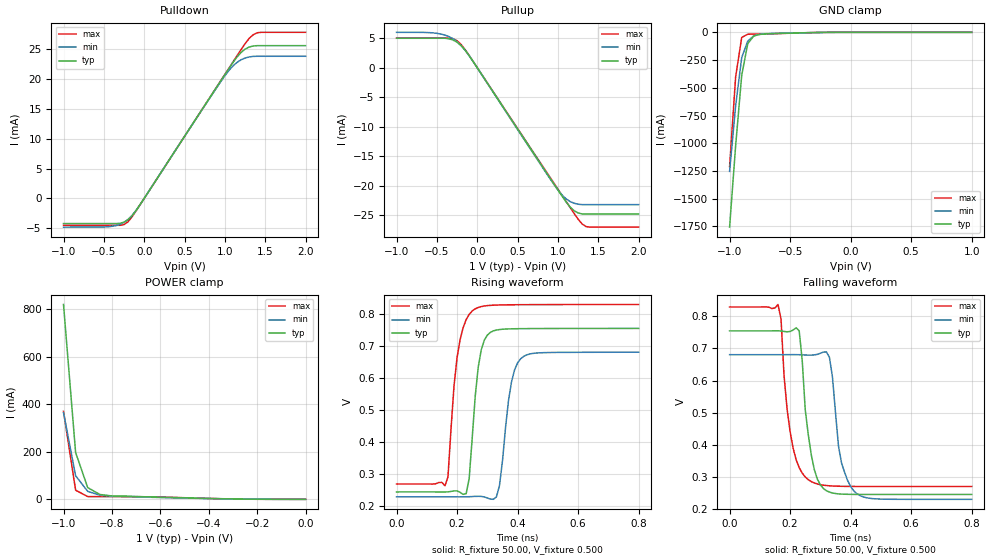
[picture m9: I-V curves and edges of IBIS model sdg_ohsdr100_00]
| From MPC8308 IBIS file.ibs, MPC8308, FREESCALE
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|Main and Boost models for Amp0: PCIx and SGMII protocols
[Model]   sdg_ohsdr100_00
Model_type 3-state
Enable Active-High
Polarity Non-Inverting
|   TYP   MIN   MAX
C_comp   0.00pF   0.00pF   0.00pF
[Model Spec]
Vmeas   0.5   0.45   0.55
[Temperature Range] 65   125   -40
[Voltage Range]   1.0   0.9   1.1
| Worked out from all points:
|   slope of the pulldown table from 0 to 0.15 V, typ, clamps not added: 48.2 ohm
|   slope of the pullup table from 0 to 0.15 V, typ, clamps not added: 48.2 ohm
|   GND clamp passes 1 mA (typ) near -0.22 V on its own axis
|   POWER clamp passes 1 mA (typ) near -0.25 V on its own axis
|   falling waveform, R_fixture 50.00, V_fixture 0.500: 20-80 % time 34ps typ, 36.1ps min, 37.8ps max; typ from 0.755 V to 0.245 V
|   rising waveform, R_fixture 50.00, V_fixture 0.500: 20-80 % time 28.6ps typ, 33.2ps min, 33.6ps max; typ from 0.245 V to 0.754 V
[Pullup]
|   Vout(V)   TYP   WCS   BCS
-1V       4.969mA    5.972mA    5.004mA
-650mV    4.969mA    5.953mA    5.004mA
-450mV    4.969mA    5.681mA    5.004mA
-300mV    4.672mA    4.885mA    4.893mA
-200mV    3.728mA    3.75mA     3.921mA
-50mV     1.018mA    1.012mA    1.029mA
950mV     -19.66mA   -19.74mA   -19.53mA
1.1V      -22.68mA   -22.18mA   -22.61mA
1.2V      -24.19mA   -22.93mA   -24.65mA
1.3V      -24.75mA   -23.17mA   -26.44mA
1.35V     -24.76mA   -23.17mA   -26.89mA
2V        -24.76mA   -23.17mA   -26.98mA
[Pulldown]
|   Vout(V)   TYP   WCS   BCS
-1V       -4.19mA    -4.788mA   -4.477mA
-400mV    -4.19mA    -4.655mA   -4.477mA
-250mV    -3.952mA   -3.99mA    -4.352mA
-200mV    -3.545mA   -3.503mA   -3.884mA
-50mV     -1.016mA   -1.002mA   -1.031mA
900mV     18.63mA    18.53mA    18.64mA
1.1V      22.7mA     22.13mA    22.78mA
1.2V      24.38mA    23.15mA    24.84mA
1.25V     24.93mA    23.44mA    25.84mA
1.35V     25.46mA    23.72mA    27.33mA
1.4V      25.51mA    23.74mA    27.66mA
2V        25.51mA    23.74mA    27.74mA
[GND Clamp]
|   Vout(V)   TYP   WCS   BCS
-1V       -1.756A    -1.253A    -1.21A
-950mV    -1.023A    -662.4mA   -401.5mA
-900mV    -388.6mA   -227.9mA   -46.1mA
-850mV    -101.9mA   -79.16mA   -16.82mA
-800mV    -32.57mA   -30.94mA   -16.19mA
-700mV    -13.95mA   -12.54mA   -14.94mA
-250mV    -1.344mA   -1.319mA   -914.3uA
1V        14.57uA    95.41uA    1.385uA
[POWER Clamp]
|   Vout(V)   TYP   WCS   BCS
-1V       820.3mA    365.3mA    370.7mA
-950mV    197mA      99.34mA    38.49mA
-900mV    49.45mA    33.55mA    11.42mA
-850mV    20.38mA    17.36mA    11.35mA
-800mV    14.23mA    12.73mA    11.26mA
-600mV    8.918mA    7.602mA    10.02mA
-300mV    1.728mA    1.566mA    1.457mA
0V        0A         0A         0A
[Falling Waveform]
R_fixture=50.00
V_fixture=0.500
V_fixture_min=0.450
V_fixture_max=0.550
|   t(s)   TYP   WCS   BCS
0s        754.7mV    680.5mV    829.1mV
160ps     754.8mV    680.5mV    836.8mV
170ps     754.4mV    680.5mV    791.7mV
190ps     751.8mV    680.5mV    511.2mV
230ps     755.1mV    680.4mV    328.7mV
260ps     431.8mV    679.2mV    291.2mV
330ps     252.5mV    672.4mV    272.1mV
370ps     246.3mV    343.3mV    270.6mV
420ps     245.3mV    248.2mV    270.1mV
800ps     245.3mV    230mV      270mV
[Rising Waveform]
R_fixture=50.00
V_fixture=0.500
V_fixture_min=0.450
V_fixture_max=0.550
|   t(s)   TYP   WCS   BCS
0s        245.3mV    230mV      270mV
160ps     245.2mV    230mV      264.3mV
200ps     248.6mV    230mV      663.8mV
230ps     239.7mV    230.1mV    781.6mV
250ps     412.4mV    230.9mV    808.7mV
290ps     717.7mV    229.7mV    824.2mV
340ps     750.9mV    264.2mV    827.4mV
380ps     753.1mV    588.2mV    828mV
410ps     753.6mV    659.7mV    828.2mV
800ps     754.5mV    680.3mV    828.8mV
[Ramp]
R_load=50.00
dV/dt_r  3.0563e-01/2.7501e-11  2.7585e-01/3.2692e-11  3.3540e-01/3.3179e-11
dV/dt_f  3.0564e-01/3.3393e-11  2.7586e-01/3.5723e-11  3.3542e-01/3.7500e-11
|[End   sdg_ohsdr100_00
